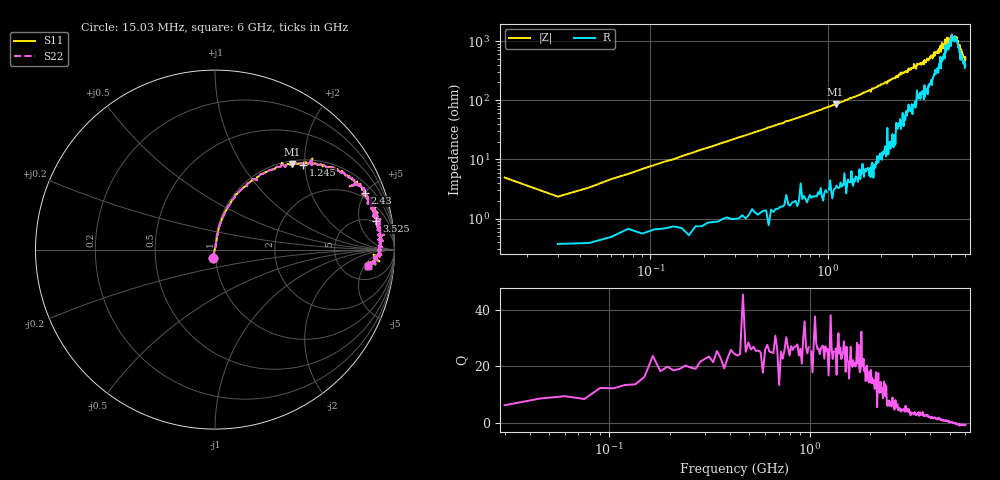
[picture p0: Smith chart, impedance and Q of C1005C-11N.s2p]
!	Network	Analyzer	HP8753E.07.74:	Oct	30	2002	Serial	No.	JP38451487
!	Hewlett-Packard
!	7	Sep	2009	8:41:45
!	Frequency	S11	S21	S12	S22
#	HZ	S	RI	R	50
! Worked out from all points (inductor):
!   400 points, 15.03 MHz to 6 GHz, reference 50 ohm
!   read as one part in series: L = 12 nH near 45.03 MHz
!   highest Q = 27.1 at 1.11 GHz (marker M1), where L = 12.3 nH
!   self-resonance near 5.197 GHz
!   S11 on the Smith chart (normalised r, x): 15.03 MHz: 0.97, -0.09; 1.245 GHz: 1.12, +1.96; 2.43 GHz: 1.61, +4.95; 3.525 GHz: 5, +9; 6 GHz: 9, -6
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1.502992e7  -0.0138 -0.0486  1.01 0.0486  1.01 0.0486  -0.0138 -0.0486
3.002985e7  0.00448 0.023  0.996 -0.023  0.996 -0.023  0.00448 0.023
6.00297e7  0.00692 0.0456  0.993 -0.0456  0.993 -0.0456  0.00692 0.0456
1.200294e8  0.0147 0.0893  0.985 -0.0893  0.985 -0.0893  0.0147 0.0893
2.850286e8  0.0518 0.2  0.948 -0.2  0.948 -0.2  0.0518 0.2
5.850271e8  0.18 0.357  0.82 -0.357  0.82 -0.357  0.18 0.357
1.020025e9  0.384 0.467  0.616 -0.467  0.616 -0.467  0.384 0.467
1.110024e9  0.427 0.476  0.573 -0.476  0.573 -0.476  0.427 0.476
1.245024e9  0.492 0.471  0.508 -0.471  0.508 -0.471  0.492 0.471
2.01002e9  0.757 0.396  0.243 -0.396  0.243 -0.396  0.757 0.396
2.430018e9  0.833 0.316  0.167 -0.316  0.167 -0.316  0.833 0.316
3.015015e9  0.894 0.236  0.106 -0.236  0.106 -0.236  0.894 0.236
3.525012e9  0.899 0.161  0.101 -0.161  0.101 -0.161  0.899 0.161
3.91501e9  0.897 0.145  0.103 -0.145  0.103 -0.145  0.897 0.145
4.00501e9  0.923 0.12  0.0768 -0.12  0.0768 -0.12  0.923 0.12
4.365008e9  0.915 0.109  0.0855 -0.109  0.0855 -0.109  0.915 0.109
4.575007e9  0.908 0.0818  0.092 -0.0818  0.092 -0.0818  0.908 0.0818
4.605007e9  0.929 0.0509  0.0709 -0.0509  0.0709 -0.0509  0.929 0.0509
5.010005e9  0.921 0.0252  0.0789 -0.0252  0.0789 -0.0252  0.921 0.0252
5.355003e9  0.927 -0.0305  0.0727 0.0305  0.0727 0.0305  0.927 -0.0305
5.625002e9  0.893 -0.0831  0.107 0.0831  0.107 0.0831  0.893 -0.0831
6e9  0.851 -0.0915  0.149 0.0915  0.149 0.0915  0.851 -0.0915
